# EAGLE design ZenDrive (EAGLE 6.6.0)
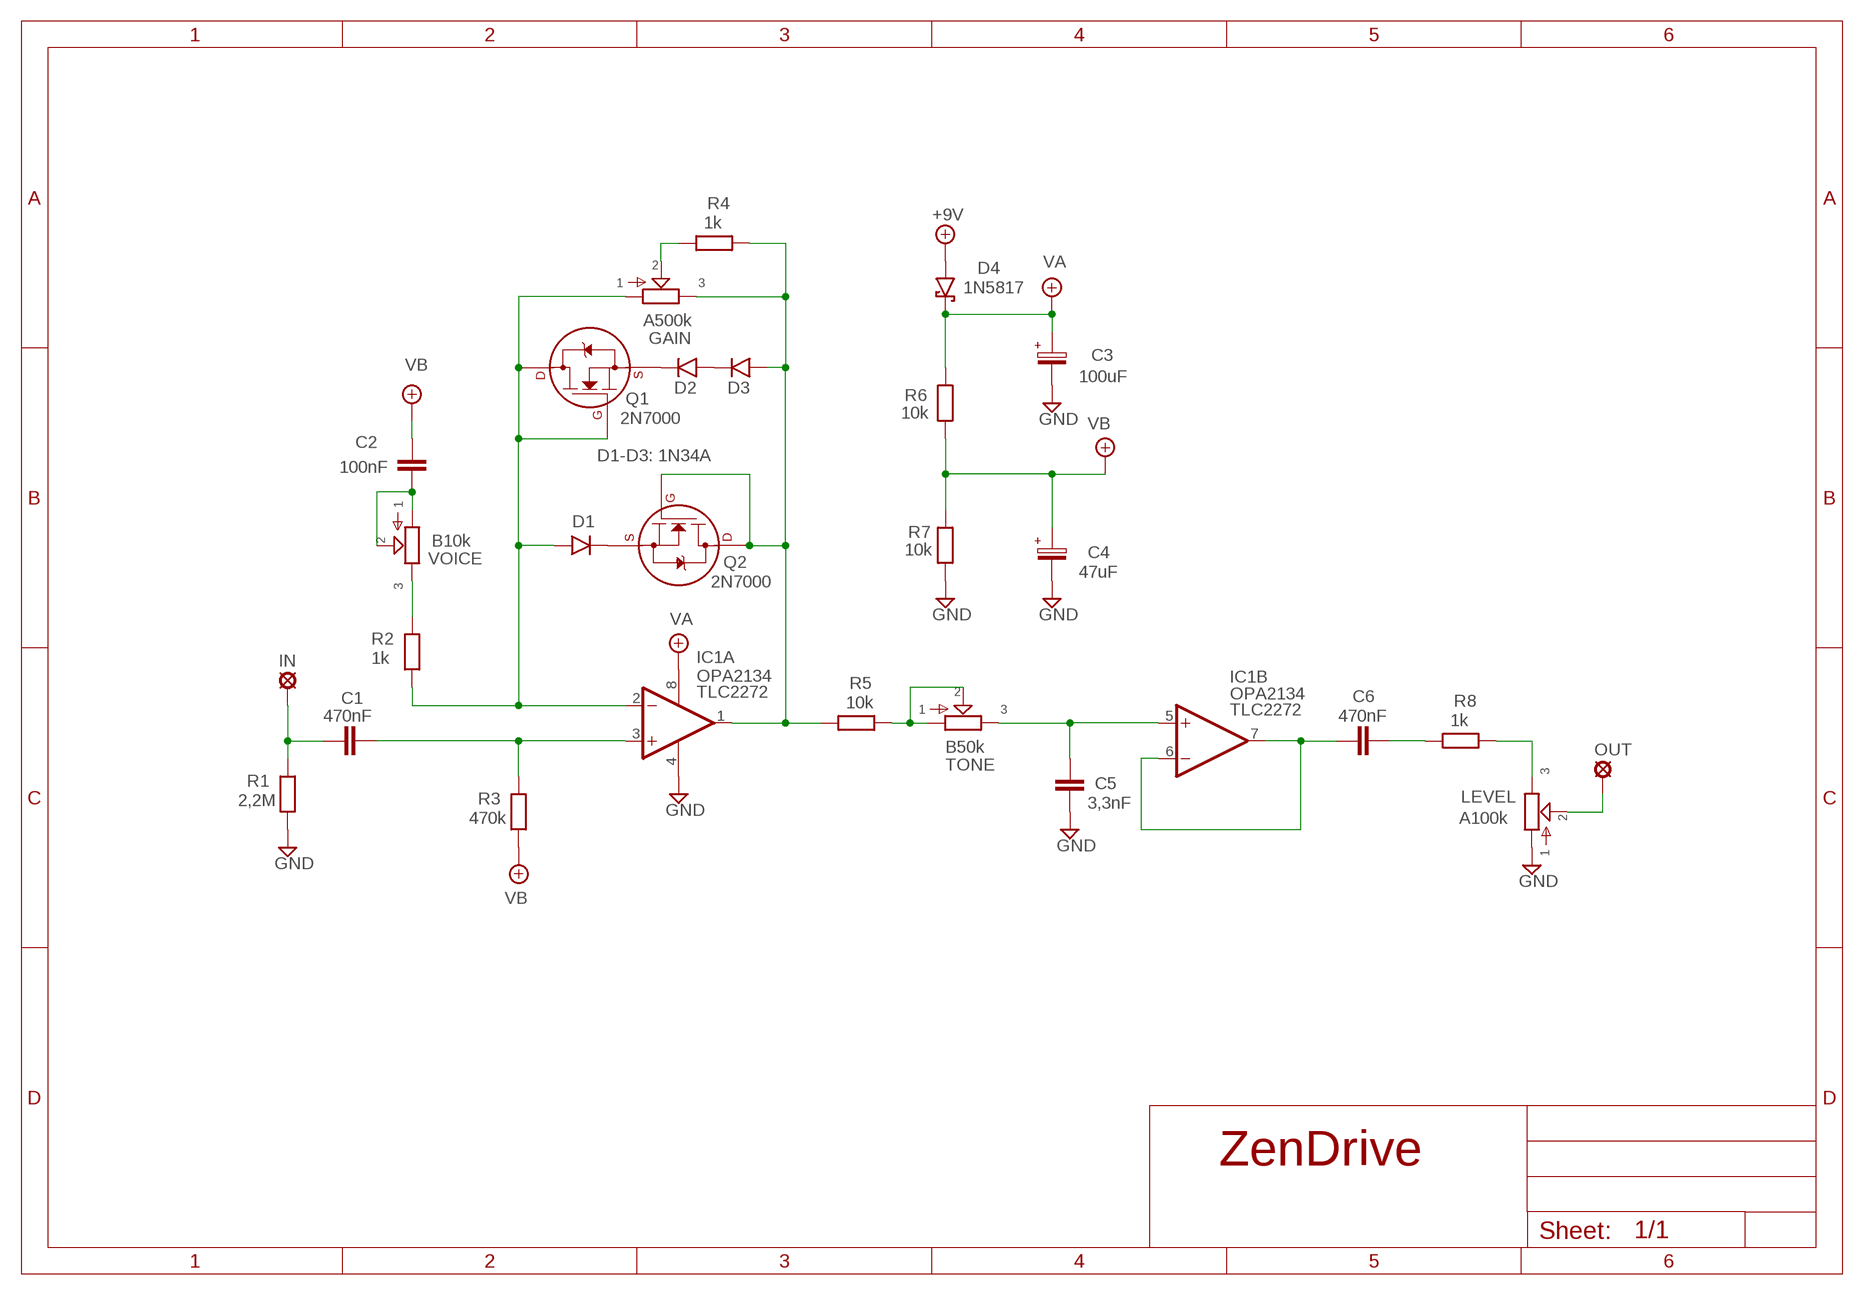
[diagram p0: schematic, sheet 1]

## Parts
+9V  +9V  +9V(T)1  [ROUND]
C1  470nF  072X0352  [072X035]
C2  100nF  072X0252  [072X025]
C3  100uF  063-EU  [063_025]
C4  47uF  063-EU  [063_025]
C5  3,3nF  072X0252  [072X025]
C6  470nF  072X0352  [072X035]
D1  DO07  [DO07]
D2  DO07  [DO07]
D3  DO07  [DO07]
D4  1N5817  [DO41-3]
GAIN  A500k  POT-EU16MM  [16MM]
GND  GND  GND(T)1  [ROUND]
GND5  GND  GND(T)1  [ROUND]
IC1  OPA2134  TL072P  [DIL08]
IN  MCS10B  [MCS10B]
LEVEL  A100k  POT-EU16MM  [16MM]
OUT  MCS10B  [MCS10B]
Q1  2N7000  2N7000_TO92  [TO-92]
Q2  2N7000  2N7000_TO92  [TO-92]
R1  2,2M  6MM-EU3  [R0207/3]
R2  1k  6MM-EU3  [R0207/3]
R3  470k  6MM-EU3  [R0207/3]
R4  1k  6MM-EU3  [R0207/3]
R5  10k  6MM-EU3  [R0207/3]
R6  10k  6MM-EU3  [R0207/3]
R7  10k  6MM-EU3  [R0207/3]
R8  1k  6MM-EU3  [R0207/3]
TONE  B50k  POT-EU16MM  [16MM]
VOICE  B10k  POT-EU16MM  [16MM]

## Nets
+9V: +9V.1(+9V) D4.A
GND: C3.- C4.- C5.2 GND5.1(GND) GND.1(GND) IC1.4(P:V-) LEVEL.1 R1.1 R7.1
N$1: C2.2 VOICE.1 VOICE.2
N$2: R2.2 VOICE.3
N$3: C1.2 IC1.3(A:+IN) R3.2
N$4: C1.1 IN.MP R1.2
N$5: D2.C Q1.1(S)
N$6: D2.A D3.C
N$7: D1.C Q2.1(S)
N$8: D1.A GAIN.1 IC1.2(A:-IN) Q1.2(G) Q1.3(D) R2.1
N$9: D3.A GAIN.3 IC1.1(A:OUT) Q2.2(G) Q2.3(D) R4.2 R5.1
N$10: GAIN.2 R4.1
N$11: C5.1 IC1.5(B:+IN) TONE.3
N$12: R5.2 TONE.1 TONE.2
N$13: C6.1 IC1.6(B:-IN) IC1.7(B:OUT)
N$14: C6.2 R8.1
N$15: LEVEL.3 R8.2
N$16: LEVEL.2 OUT.MP
VA: C3.+ D4.C IC1.8(P:V+) R6.2
VB: C2.1 C4.+ R3.1 R6.1 R7.2

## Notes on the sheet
- D1-D3: 1N34A
- TLC2272
- TLC2272

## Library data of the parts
+9V = gm-supply:+9V(T): +9V Voltage Supply
C1 C6 = Wima MKS:072X035: 0.15 - 1.0uF;
C2 C5 = Wima MKS:072X025: 1000pF - 0.47uF
C3 C4 = Elektrolyytit:063-EU
D1-D3 = gm-diodes:DO07: DO-07 Package
D4 = Diodit:1N5817
GAIN LEVEL TONE VOICE = gm-pots:POT-EU
GND GND5 = gm-supply:GND(T): Ground
IC1 = Operaatiovahvistimet:TL072: OP AMP
IN OUT = Padit:MCS10B: SOLDER PAD
Q1 Q2 = transistors:2N700*: 2N7000, 2N7002, NDS7002A N-channel enhancement mode MOSFET
R1-R8 = Vastukset:6MM-EU: 6mm Resistors (European schematic symbol)

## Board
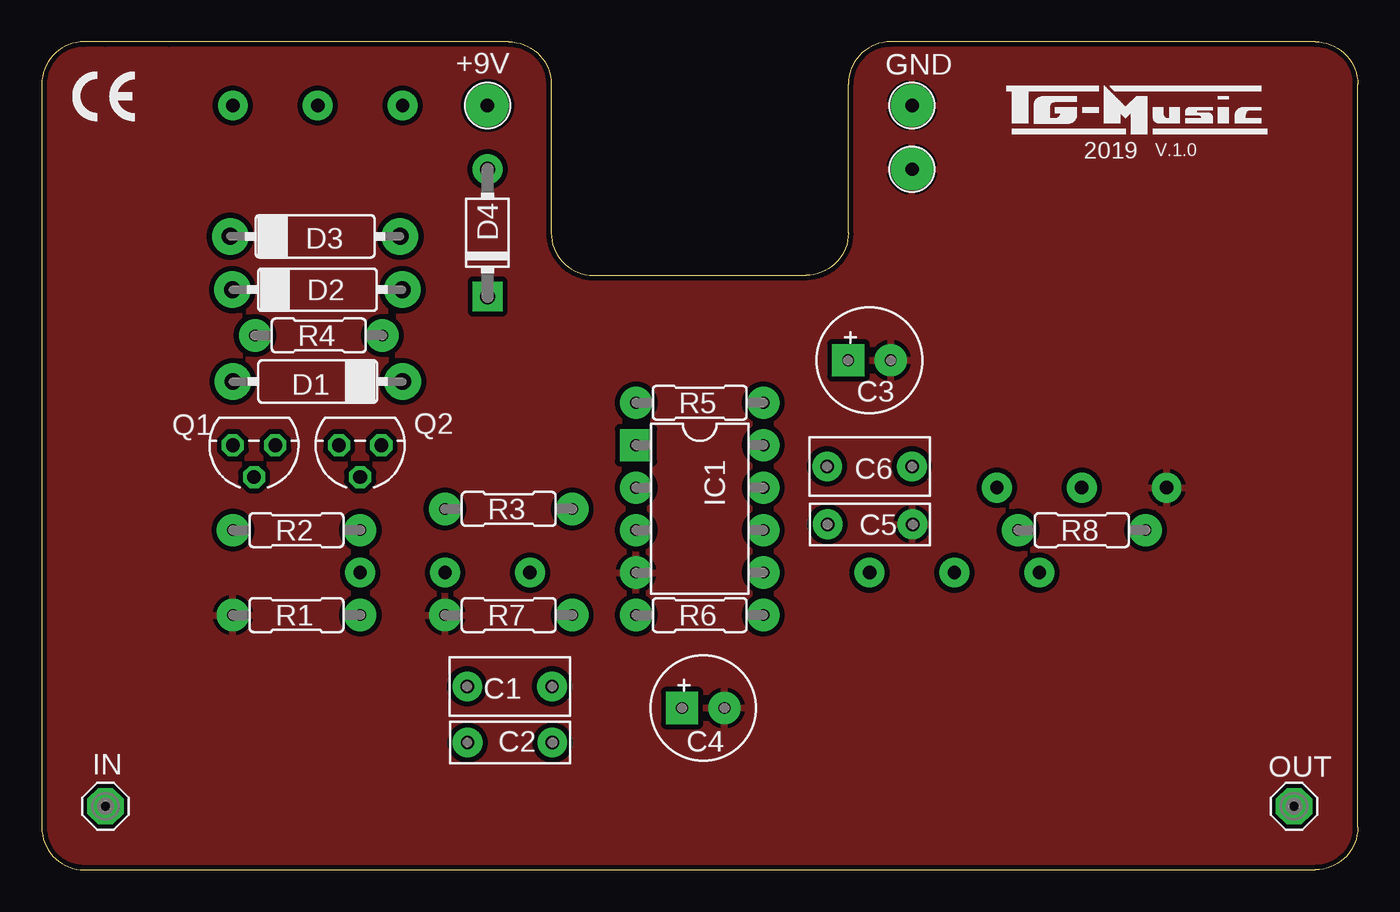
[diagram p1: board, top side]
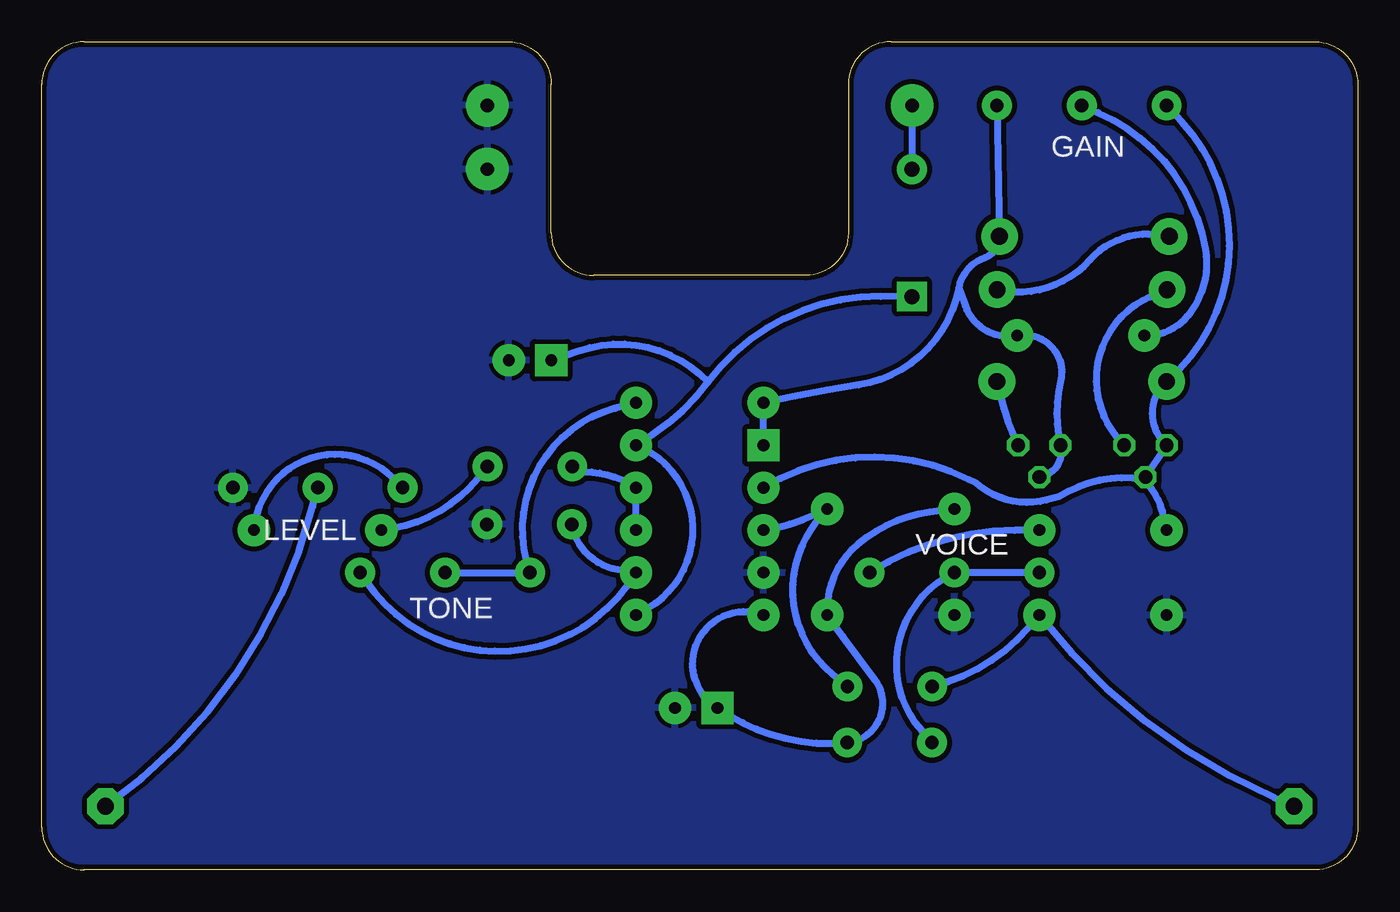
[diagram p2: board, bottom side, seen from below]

Size 78.74 x 49.53 mm. Coordinates in mm from the lower left corner, seen from the top.
Outline: 7.62,49.53 3.81,49.53
Outline: 78.74,2.54 78.74,46.99 arc90 76.2,49.53 50.8,49.53 arc90 48.26,46.99 48.26,38.1 arc-90 45.72,35.56 33.02,35.56 arc-90 30.48,38.1 30.48,46.99 arc90 27.94,49.53 2.54,49.53 arc90 0,46.99 0,2.54 arc90 2.54,0 76.2,0 arc90 78.74,2.54
Copper layers (1*16): Top 0.035mm / dielectric 1.5mm / Bottom 0.035mm
Design rules "ITEADstudio": minimum track width 10mil, minimum drill 12mil, track to track 12mil, track to pad 12mil, pad to pad 12mil, via to via 12mil, smd to smd 0mil, copper to edge 12mil, drill to drill 12mil, minimum pad ring 10mil, minimum via ring 6mil, stop-mask expansion 4mil, vias tented up to drill 100mil, thermal gap 10mil

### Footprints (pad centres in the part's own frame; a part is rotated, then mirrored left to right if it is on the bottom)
ROUND = drill 0.8 pad 2.54: 1 0,0
072X035 = drill 0.8 pad 1.778: 1 -2.54,0; 2 2.54,0
072X025 = drill 0.8 pad 1.778: 1 -2.54,0; 2 2.54,0
063_025 = drill 0.7 pad 1.93 square: + -1.27,0 | drill 0.7 pad 1.93: - 1.27,0
DO07 = drill 1 pad 2.184: A 5.08,0; C -5.08,0
DO41-3 = drill 0.9 pad 1.778: A 3.81,0 | drill 0.9 pad 1.778 square: C -3.81,0
16MM = drill 0.8 pad 1.778: 1 5.08,0; 2 0,0; 3 -5.08,0
DIL08 = drill 0.7 pad 1.93 square: 1 -3.81,-3.81 | drill 0.7 pad 1.93: 2 -1.27,-3.81; 3 1.27,-3.81; 4 3.81,-3.81; 5 3.81,3.81; 6 1.27,3.81; 7 -1.27,3.81; 8 -3.81,3.81
MCS10B = drill 1.016 pad 2.159 octagon: MP 0,0
TO-92 = drill 0.813 octagon: 1 -1.27,0; 2 0,1.905; 3 1.27,0
R0207/3 = drill 0.7 pad 1.93: 1 -3.81,0; 2 3.81,0

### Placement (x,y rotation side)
+9V  26.67,45.72 0 top
C1  28,10.97 0 top
C2  28.01,7.61 180 top
C3  49.53,30.48 0 top
C4  39.58,9.68 0 top
C5  49.56,20.67 0 top
C6  49.53,24.13 0 top
D1  16.51,29.21 180 top
D2  16.49,34.7 0 top
D3  16.36,37.89 0 top
D4  26.67,38.1 90 top
GAIN  16.51,45.72 0 bottom
GND  52.07,45.72 0 top
GND5  52.07,41.91 0 top
IC1  39.37,21.59 270 top
IN  3.81,3.81 0 top
LEVEL  62.23,22.86 180 bottom
OUT  74.93,3.81 0 top
Q1  12.7,25.4 180 top
Q2  19.05,25.4 180 top
R1  15.24,15.24 0 top
R2  15.24,20.32 0 top
R3  27.94,21.59 0 top
R4  16.57,31.97 0 top
R5  39.37,27.94 0 top
R6  39.37,15.24 0 top
R7  27.94,15.24 0 top
R8  62.23,20.32 0 top
TONE  54.61,17.78 0 bottom
VOICE  24.13,17.78 0 bottom

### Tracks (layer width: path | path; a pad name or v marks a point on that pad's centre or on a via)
+9V
  Bottom 0.406: +9V.1 D4.A
GND
  pour Bottom: 0,2.54 0,46.99 arc-90 2.54,49.53 27.94,49.53 arc-90 30.48,46.99 30.48,38.1 arc90 33.02,35.56 45.72,35.56 arc90 48.26,38.1 48.26,46.99 arc-90 50.8,49.53 76.2,49.53 arc-90 78.74,46.99 78.74,2.54 arc-90 76.2,0 2.54,0 arc-90
  pour Top: 0,2.54 0,46.99 arc-90 2.54,49.53 27.94,49.53 arc-90 30.48,46.99 30.48,38.1 arc90 33.02,35.56 45.72,35.56 arc90 48.26,38.1 48.26,46.99 arc-90 50.8,49.53 76.2,49.53 arc-90 78.74,46.99 78.74,2.54 arc-90 76.2,0 2.54,0 arc-90
N$1
  Bottom 0.406: VOICE.1 VOICE.2 arc-106 26.09,8.31 C2.2
N$2
  Bottom 0.406: R2.2 20.52,20.31 arc-31 VOICE.3
N$3
  Bottom 0.406: IC1.3 arc-19 R3.2 arc-20 33.22,19.41 arc-75 31.41,11.69 C1.2
N$4
  Bottom 0.406: C1.1 arc-36 19.73,14.46 R1.2 arc-29 4.99,4.32 IN.MP
N$5
  Bottom 0.406: D2.C 12.39,34.28 arc-113 Q1.1
N$6
  Bottom 0.406: D3.C 12.09,37.99 arc-55 16.02,36.48 arc61 D2.A
N$7
  Bottom 0.406: D1.C 21.38,28.34 arc-13 Q2.1
N$8
  Bottom 0.406: GAIN.1 10.57,44.78 arc92 D1.A arc-98 Q1.3 Q1.2 12.83,23.37 | 12.83,23.37 arc-40 17.87,22.32 18.6,22.13 arc56 22.81,23.11 23.28,23.35 arc-58 IC1.2 | R2.1 11.59,21.1 arc-34 12.83,23.37
N$9
  Bottom 0.406: GAIN.3 D3.A arc72 22.33,36.6 arc-60 23.87,34.8 | IC1.1 R5.1 arc4 29.86,29.01 arc-71 23.87,34.8 | 23.87,34.8 23.49,33.74 arc-81 R4.2 arc114 17.78,29.21 arc-28 Q2.3 arc95 Q2.2
N$10
  Bottom 0.406: GAIN.2 15.54,45.3 arc57 9.12,37.12 arc45 9.97,33.39 arc42 12.15,31.96 R4.1
N$11
  Bottom 0.406: C5.1 arc-71 44.27,17.96 IC1.5 arc116 59.39,17.33 TONE.3
N$12
  Bottom 0.406: TONE.2 TONE.1 arc95 44.44,27.6 R5.2
N$13
  Bottom 0.406: IC1.6 IC1.7 arc-34 46.3,23.8 46.66,23.8 C6.1
N$14
  Bottom 0.406: C6.2 52.67,23.39 arc45 R8.1
N$15
  Bottom 0.406: LEVEL.3 57.7,23.41 arc-131 R8.2
N$16
  Bottom 0.406: OUT.MP arc-40 62.52,21.75 LEVEL.2
VA
  Bottom 0.406: R6.2 42.46,15.66 arc-128 IC1.8 arc-24 38.87,29.2 | D4.C 28.55,34.3 arc-54 38.87,29.2 | C3.+ 46.61,31.05 arc65 38.87,29.2
VB
  Bottom 0.406: R3.1 25.6,21.39 arc-32 29.91,19.48 arc-53 R7.2 arc0 28.88,11.36 arc121 C2.1 arc37 37.6,9.25 C4.+ arc169 R6.1

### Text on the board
tNames: 2019 | V.1.0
